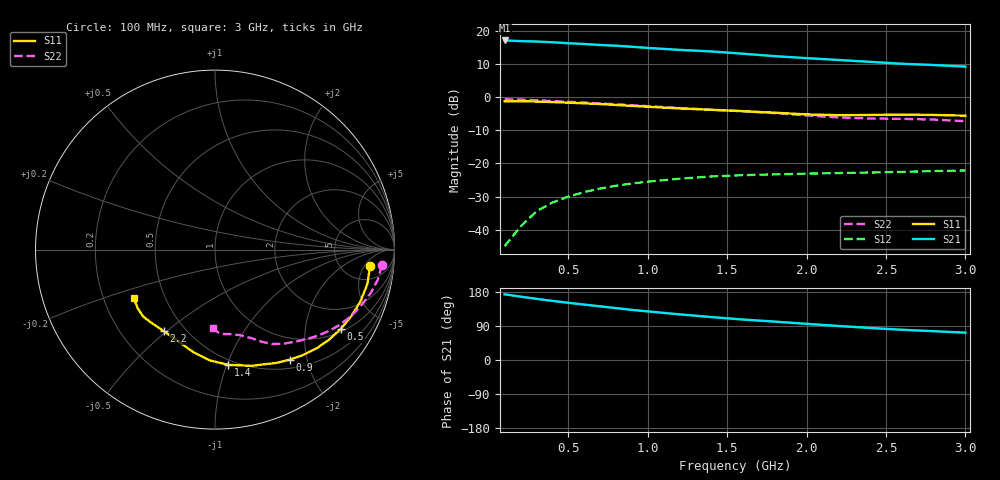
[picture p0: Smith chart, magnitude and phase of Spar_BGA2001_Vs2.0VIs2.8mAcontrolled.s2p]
! Filename: 22_8G1.001
! Title: BGA2001 X0297-20 HFE=80
! Bias: Vce=2V; Ic=2.8mA controlled / noise data included
! Company: NXP Semiconductors NL
! User: Quality&Reliability T&D
! Measure time: 23 Oct 1998 / 08:33:35
#  MHz  S  MA  R 50
! Freq  S11  S21  S12  S22  :
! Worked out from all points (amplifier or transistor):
!   20 points, 100 MHz to 3 GHz, reference 50 ohm
!   highest |S21| = 17.2 dB at 100 MHz (marker M1)
!   |S21| within 3 dB of that: start of sweep to 1.267 GHz
!   unconditionally stable (mu >= 1): 2.544 GHz to end of sweep
!   at 400 MHz: K = 0.18, MSG = 24.2 dB, |S12| = -31.8 dB
!   at 1.2 GHz: K = 0.44, MSG = 19.5 dB, |S12| = -24.6 dB
!   at 3 GHz: K = 1.17, MAG = 13.2 dB, |S12| = -22.1 dB
!   lowest NFmin = 1.13 dB at 1.8 GHz
!   S11 on the Smith chart (normalised r, x): 100 MHz: 9, -7; 500 MHz: 1.10, -3.11; 900 MHz: 0.63, -1.71; 1.4 GHz: 0.46, -1.01; 2.2 GHz: 0.38, -0.49; 3 GHz: 0.33, -0.25
100  0.8686 -6.2  7.208 173.3  0.005642 59.8  0.934 -5.4
200  0.8704 -12.6  7.05 167.3  0.01113 81.8  0.9221 -10.5
300  0.8605 -19.4  6.942 161.4  0.01894 79.8  0.9015 -15.5
400  0.8452 -26.0  6.774 156.0  0.02566 75.3  0.8768 -19.9
500  0.8287 -32.2  6.544 151.0  0.03155 71.5  0.8554 -24.0
600  0.8095 -38.3  6.375 146.2  0.03696 67.9  0.8313 -27.9
700  0.7895 -44.1  6.156 141.6  0.04176 64.6  0.8084 -31.5
800  0.7654 -50.1  6.007 137.0  0.04612 61.5  0.7839 -35.0
900  0.7416 -55.8  5.791 132.4  0.04979 58.7  0.759 -38.3
1000  0.7188 -61.4  5.561 128.3  0.05313 56.3  0.7344 -41.6
1200  0.6785 -72.7  5.198 120.5  0.05888 52.0  0.6873 -47.9
1400  0.6463 -83.5  4.919 113.3  0.06366 48.4  0.6493 -53.8
1600  0.6173 -92.9  4.549 106.8  0.06663 46.1  0.6146 -58.9
1800  0.5846 -101.8  4.176 101.3  0.0685 45.1  0.5761 -63.1
2000  0.5517 -111.5  3.9 95.4  0.07025 43.3  0.5323 -67.8
2200  0.5364 -121.9  3.659 89.8  0.0717 41.7  0.4963 -73.8
2400  0.5403 -130.7  3.426 84.5  0.07307 41.2  0.4776 -80.2
2600  0.5473 -137.2  3.207 79.9  0.07463 42.3  0.4721 -85.1
2800  0.5404 -142.9  3.067 76.0  0.07688 42.4  0.4603 -88.2
3000  0.5273 -149.3  2.906 72.1  0.07847 43.2  0.4349 -91.5
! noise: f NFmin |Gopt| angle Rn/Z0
900  1.19  0.43  19  0.33
1000  1.22  0.42  18  0.32
1800  1.134  0.398  62.94  0.265
2000  1.181  0.359  74.05  0.262
2200  1.384  0.299  83.76  0.228
2400  1.525  0.289  94.61  0.217
